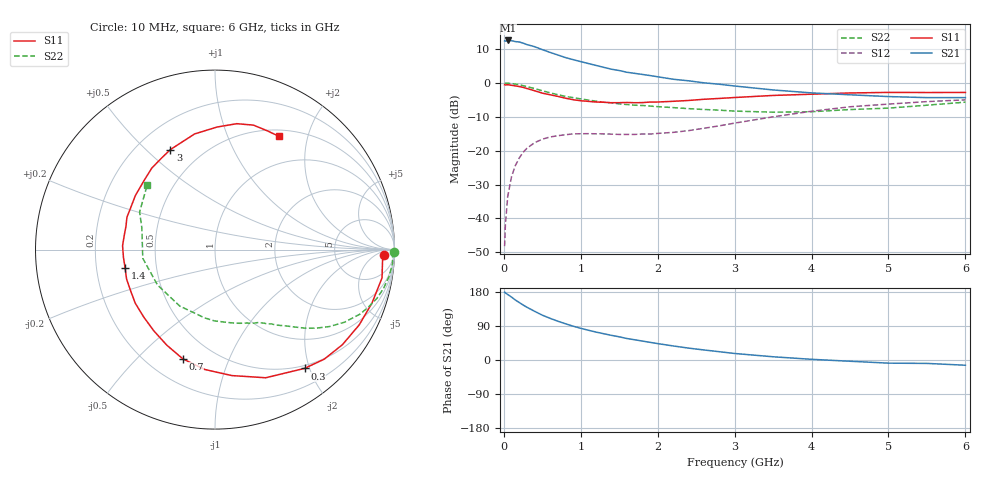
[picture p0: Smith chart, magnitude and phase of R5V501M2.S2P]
! SIEMENS Small Signal Semiconductors
! BFR183
! Si NPN RF Bipolar Junction Transistor in SOT23
! VCE = 0.5 V  IC = 1.2 mA
! Common Emitter S-Parameters:  May  1996
# GHz  S  MA  R  50
!  f  S11  S21  S12  S22
! GHz  MAG  ANG  MAG  ANG  MAG  ANG  MAG  ANG
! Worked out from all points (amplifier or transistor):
!   36 points, 10 MHz to 6 GHz, reference 50 ohm
!   highest |S21| = 12.6 dB at 50 MHz (marker M1)
!   |S21| within 3 dB of that: start of sweep to 536.3 MHz
!   unconditionally stable (mu >= 1): 1.498 GHz to 3.859 GHz; 5.236 GHz to end of sweep
!   at 250 MHz: K = 0.19, MSG = 16.1 dB, |S12| = -20.5 dB
!   at 1.4 GHz: K = 0.95, MSG = 9.6 dB, |S12| = -15.1 dB
!   at 6 GHz: K = 1.01, MAG = -0.2 dB, |S12| = -5.0 dB
!   S11 on the Smith chart (normalised r, x): 10 MHz: 26, -15; 300 MHz: 0.45, -1.92; 700 MHz: 0.34, -0.69; 1.4 GHz: 0.33, -0.09; 3 GHz: 0.34, +0.60; 6 GHz: 0.58, +1.55
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0.01  0.9428 -1.9  4.178 179.1  0.0039 88.6  0.9958 -0.8
0.02  0.9355 -3.8  4.139 177.1  0.008 87.5  0.9899 -1.7
0.05  0.9438 -9.6  4.243 172.9  0.021 84.0  0.9919 -4.4
0.1  0.9241 -18.8  4.217 166.0  0.0414 79.0  0.9816 -8.7
0.15  0.9063 -27.6  4.081 158.3  0.0605 73.0  0.9635 -13.0
0.2  0.8859 -36.7  4.03 151.7  0.0779 68.0  0.9419 -16.8
0.25  0.862 -45.1  3.875 145.2  0.0945 63.2  0.9125 -20.6
0.3  0.8287 -53.0  3.688 139.2  0.1087 58.8  0.884 -24.0
0.4  0.7679 -68.4  3.434 128.5  0.1314 51.3  0.8269 -29.3
0.5  0.7081 -82.4  3.107 118.3  0.1481 44.7  0.7686 -33.9
0.6  0.6703 -94.9  2.831 110.1  0.1593 39.5  0.7164 -37.6
0.7  0.6345 -106.4  2.595 102.5  0.1665 35.3  0.6723 -40.7
0.9  0.5666 -127.0  2.212 89.3  0.1771 29.2  0.6075 -45.0
1.1  0.5354 -146.0  1.935 78.5  0.1785 25.4  0.5593 -49.1
1.4  0.5111 -168.5  1.596 65.0  0.1756 23.4  0.5072 -54.8
1.8  0.5129 165.3  1.338 50.0  0.1763 26.9  0.4652 -61.6
2.2  0.5363 145.7  1.136 37.1  0.1866 33.1  0.4332 -71.4
3  0.6103 114.0  0.902 17.2  0.2556 40.1  0.3844 -98.8
3.5  0.6544 100.0  0.789 8.5  0.3165 37.9  0.3709 -122.0
4.5  0.712 80.2  0.669 -3.3  0.4453 25.5  0.4053 -173.1
5.5  0.7231 66.2  0.608 -9.0  0.5309 11.4  0.4697 153.4
6  0.7245 60.7  0.608 -13.8  0.5637 2.7  0.521 136.5
